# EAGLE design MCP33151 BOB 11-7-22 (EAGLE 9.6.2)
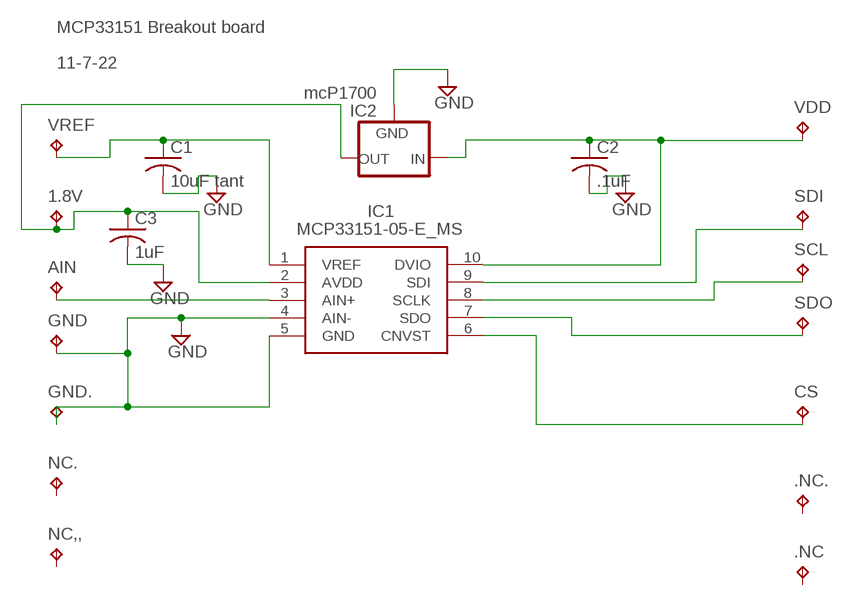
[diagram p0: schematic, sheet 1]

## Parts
1.8V  TPPAD1-13  [P1-13]
.NC  TPPAD1-13  [P1-13]
.NC.  TPPAD1-13  [P1-13]
AIN  TPPAD1-13  [P1-13]
C1  10uF tant  C-USC1206  [C1206]
C2  .1uF  C-USC1206  [C1206]
C3  1uF  C-USC1206  [C1206]
CS  TPPAD1-13  [P1-13]
GND  TPPAD1-13  [P1-13]
GND.  TPPAD1-13  [P1-13]
IC1  MCP33151-05-E_MS  [SOP50P490X110-10N]
IC2  mcP1700  MCP1700INLINE  [TO92-INLINE]
NC,,  TPPAD1-13  [P1-13]
NC.  TPPAD1-13  [P1-13]
SCL  TPPAD1-13  [P1-13]
SDI  TPPAD1-13  [P1-13]
SDO  TPPAD1-13  [P1-13]
VDD  TPPAD1-13  [P1-13]
VREF  TPPAD1-13  [P1-13]

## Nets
GND: C1.2 C2.2 C3.2 GND..TP GND.TP IC1.4(AIN-) IC1.5(GND) IC2.1(GND)
N$1: C1.1 IC1.1(VREF) VREF.TP
N$2: AIN.TP IC1.3(AIN+)
N$3: C2.1 IC1.10(DVIO) IC2.2(IN) VDD.TP
N$4: IC1.9(SDI) SDI.TP
N$5: IC1.8(SCLK) SCL.TP
N$6: IC1.7(SDO) SDO.TP
N$7: CS.TP IC1.6(CNVST)
N$8: 1.8V.TP C3.1 IC1.2(AVDD) IC2.3(OUT)
Unconnected: .NC..TP .NC.TP NC,,.TP NC..TP

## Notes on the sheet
- MCP33151 Breakout board
- 11-7-22

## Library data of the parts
1.8V .NC .NC. AIN CS GND GND. NC,, NC. SCL SDI SDO VDD VREF = testpad:TP: Test pad
C1-C3 = adafruit:C-US: CAPACITOR, American symbol
IC1 = MCP33151-05-E_MS:MCP33151-05-E_MS: Analog to Digital Converters - ADC 14-bit, 500 ksps, single channel, single-ended SAR ADC Source: Datasheet; DESCRIPTION: Analog to Digital Converters - ADC 14-bit, 500 ksps, single channel, single-ended SAR ADC; HEIGHT: 1.1mm; MANUFACTURER_NAME: Microchip; MANUFACTURER_PART_NUMBER: MCP33151-05-E/MS; MOUSER_PART_NUMBER: 579-MCP33151-05-E/MS; MOUSER_PRICE-STOCK: https://www.mouser.co.uk/ProductDetail/Microchip-Technology/MCP33151-05-E-MS?qs=T3oQrply3y%252BD0A%2FnRLKX1g%3D%3D
IC2 = adafruit:MCP1700: VOLTAGE REGULATOR

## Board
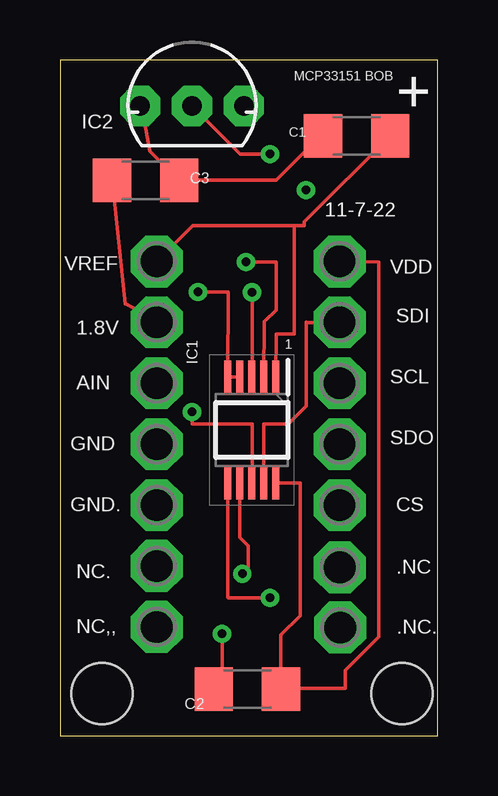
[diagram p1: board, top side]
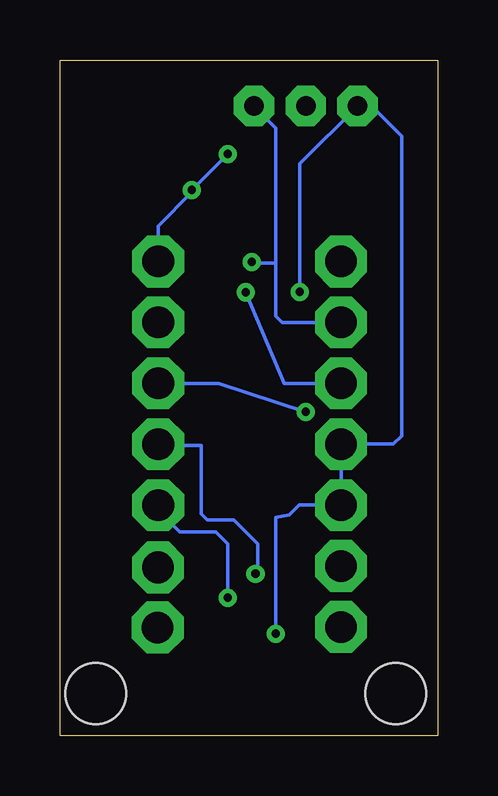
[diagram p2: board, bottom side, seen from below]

Size 15.74 x 28.17 mm. Coordinates in mm from the lower left corner, seen from the top.
Outline: 0,0 15.74,0 15.74,28.17 0,28.17 0,0
Copper layers (1*16): Top 0.035mm / dielectric 1.5mm / Bottom 0.035mm
Design rules "default": minimum track width 6mil, minimum drill 0.35mm, track to track 6mil, track to pad 6mil, pad to pad 6mil, via to via 6mil, smd to smd 6mil, copper to edge 40mil, drill to drill 6mil, minimum pad ring 10mil, minimum via ring 8mil, stop-mask expansion 4mil, vias tented up to drill 0mil, thermal gap 10mil
Holes 2.54 mm at 1.75,1.75 14.25,1.75

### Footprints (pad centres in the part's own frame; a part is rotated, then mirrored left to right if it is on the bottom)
P1-13 = drill 1.321 pad 2.159 octagon: TP 0,0
C1206 = smd 1.6 x 1.8: 1 -1.4,0; 2 1.4,0
SOP50P490X110-10N = smd 1.4 x 0.3: 1 -2.2,1; 2 -2.2,0.5; 3 -2.2,0; 4 -2.2,-0.5; 5 -2.2,-1; 6 2.2,-1; 7 2.2,-0.5; 8 2.2,0; 9 2.2,0.5; 10 2.2,1
TO92-INLINE = drill 0.813 pad 1.676 octagon: 1 -2.159,0; 2 0,0; 3 2.159,0

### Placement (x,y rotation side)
1.8V  4.03,17.23 0 top
.NC  11.66,7.01 0 top
.NC.  11.67,4.51 0 top
AIN  4.03,14.69 0 top
C1  12.36,25 180 top
C2  7.81,1.94 180 top
C3  3.57,23.15 0 top
CS  11.65,9.61 0 top
GND  4.03,12.15 0 top
GND.  4.03,9.61 0 top
IC1  7.99,12.74 270 top
IC2  5.5,26.25 0 top
NC,,  4.03,4.53 0 top
NC.  4.03,7.07 0 top
SCL  11.65,14.69 0 top
SDI  11.65,17.23 0 top
SDO  11.65,12.15 0 top
VDD  11.65,19.77 0 top
VREF  4.03,19.77 0 top

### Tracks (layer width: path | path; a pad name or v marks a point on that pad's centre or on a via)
GND  (via drill 0.35)
  Top 0.152: C2.2 6.75,2.28 v6.75,4.25 | v5.75,18.5 7.01,18.5 IC1.5 IC1.4 | IC2.1 3.4,26.24 3.74,24.38 C3.2 9,23.15 10.85,25 C1.2
  Bottom 0.152: v6.75,4.25 6.75,9.09 6.19,9.2 5.78,9.61 GND..TP GND.TP 1.85,12.15 1.5,12.5 1.5,25 2.75,26.25 IC2.1 5.75,23.84 v5.75,18.5
N$1
  Top 0.152: IC1.1 9,16.75 9.75,16.75 9.75,21.27 | C1.1 10.19,21.43 10.18,21.27 9.75,21.27 | VREF.TP 5.53,21.27 9.75,21.27
N$2  (via drill 0.35)
  Top 0.152: IC1.3 8.02,14.97 v8,18.48
  Bottom 0.152: AIN.TP 6.39,14.69 v8,18.48
N$3  (via drill 0.35)
  Top 0.152: VDD.TP 11.5,19.77 13.28,19.75 13.28,4.12 11.89,2.73 11.89,1.98 9.53,1.98 9.39,2.11 C2.1 9.21,4.21 10,5 10,10.54 IC1.10 | v8.75,24.25 7.5,24.25 IC2.2
  Bottom 0.152: VDD.TP 11.65,21.25 10.25,22.65 v10.25,22.75 v8.75,24.25
N$4
  Top 0.152: SDI.TP 10.35,17.23 10.25,17.25 10.25,13.75 9.5,13 8.49,13 IC1.9
N$5  (via drill 0.35)
  Top 0.152: IC1.8 8,12 8,13 5.5,13 v5.5,13.5
  Bottom 0.152: SCL.TP 9.12,14.69 v5.5,13.5
N$6  (via drill 0.35)
  Top 0.152: v7.6,6.75 7.85,7 7.85,7.9 7.49,8.26 IC1.7
  Bottom 0.152: SDO.TP 11.6,12.11 9.86,12.11 9.86,9.25 9.61,9 8.5,9 7.5,8 7.5,6.75 v7.6,6.75
N$7  (via drill 0.35)
  Top 0.152: IC1.6 6.99,5.76 7,5.75 v8.75,5.75
  Bottom 0.152: CS.TP 11.65,9.4 10.75,8.5 9.25,8.5 8.75,8 v8.75,5.75
N$8  (via drill 0.35)
  Top 0.152: IC1.2 8.51,17.26 9,17.75 9,19.75 v7.75,19.75 | 1.8V.TP 3.9,17.36 2.75,18 2.73,18 C3.1
  Bottom 0.152: IC2.3 6.74,25.34 6.74,19.71 | 1.8V.TP 6.48,17.23 6.74,17.49 6.74,19.71 | v7.75,19.75 7.71,19.71 6.74,19.71

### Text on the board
tNames: MCP33151 BOB | + | 11-7-22 | 1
